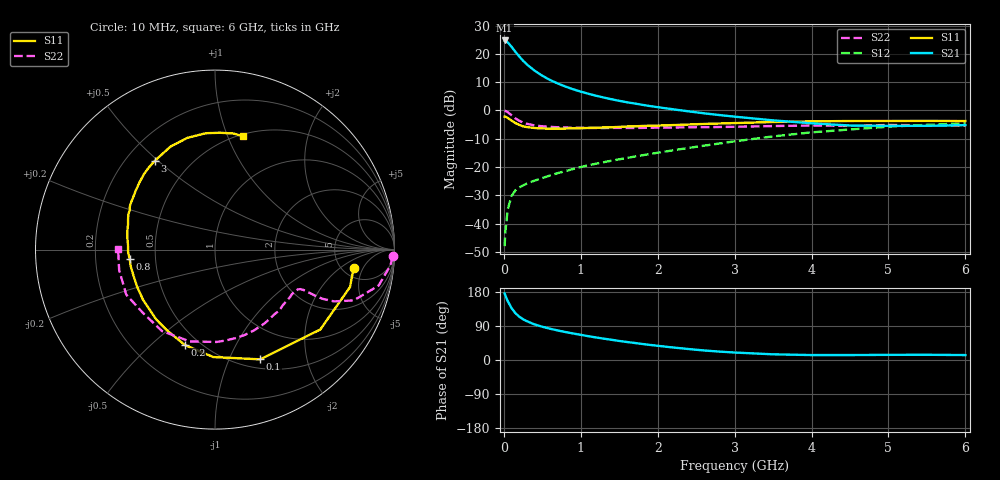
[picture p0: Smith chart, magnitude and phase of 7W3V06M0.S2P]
! Infineon Technologies  Discrete & RF Semiconductors
! BFS17W
! Si NPN RF Bipolar Junction Transistor in SOT323
! VCE = 3 V  IC = 6 mA
! Common Emitter S-Parameters:  August  1999
# GHz  S  MA  R  50
!  f  S11  S21  S12  S22
! GHz  MAG  ANG  MAG  ANG  MAG  ANG  MAG  ANG
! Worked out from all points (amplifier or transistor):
!   36 points, 10 MHz to 6 GHz, reference 50 ohm
!   highest |S21| = 24.7 dB at 10 MHz (marker M1)
!   |S21| within 3 dB of that: start of sweep to 121.7 MHz
!   unconditionally stable (mu >= 1): 499.1 MHz to 2.805 GHz; 4.255 GHz to end of sweep
!   at 250 MHz: K = 0.65, MSG = 22.0 dB, |S12| = -26.5 dB
!   at 1.4 GHz: K = 1.24, MAG = 7.9 dB, |S12| = -17.8 dB
!   at 6 GHz: K = 1.08, MAG = -2.1 dB, |S12| = -4.5 dB
!   S11 on the Smith chart (normalised r, x): 10 MHz: 6.29, -3.30; 100 MHz: 0.60, -1.31; 200 MHz: 0.42, -0.64; 800 MHz: 0.35, -0.05; 3 GHz: 0.32, +0.49; 6 GHz: 0.52, +1.14
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0.01  0.7791 -7.6  17.24 175.4  0.004 79.9  0.9921 -2.2
0.02  0.7807 -15.5  17.04 169.9  0.0072 85.0  0.9805 -5.3
0.05  0.7365 -37.2  16.02 155.6  0.0178 73.5  0.9333 -12.4
0.1  0.6613 -67.6  13.33 137.1  0.0307 60.7  0.8235 -20.1
0.15  0.5986 -91.0  10.88 123.6  0.0387 53.4  0.7237 -23.5
0.2  0.5571 -107.6  8.994 114.4  0.0435 51.5  0.6583 -24.6
0.25  0.5242 -120.3  7.559 107.6  0.0475 49.0  0.6105 -24.7
0.3  0.5082 -130.2  6.491 102.3  0.0511 49.3  0.5813 -24.6
0.4  0.4889 -145.1  5.043 93.9  0.0576 50.7  0.543 -24.5
0.5  0.4805 -154.8  4.104 87.8  0.0638 52.9  0.5248 -24.8
0.6  0.4767 -162.6  3.453 82.6  0.0709 54.7  0.513 -25.6
0.8  0.4783 -173.9  2.646 73.8  0.0847 57.7  0.4991 -28.6
0.9  0.4845 -178.4  2.368 70.0  0.0923 59.4  0.4949 -30.4
1.1  0.4905 173.6  1.969 62.7  0.1076 61.0  0.4919 -34.6
1.3  0.5009 166.7  1.69 56.3  0.1221 62.3  0.4888 -39.6
1.6  0.5212 158.0  1.395 47.5  0.1446 63.7  0.4895 -47.3
2.2  0.5512 143.1  1.047 33.0  0.1977 65.5  0.5001 -64.5
3  0.5981 124.0  0.777 19.7  0.2843 63.4  0.5146 -89.0
3.5  0.6254 113.3  0.668 15.0  0.3482 59.6  0.5304 -105.3
4.5  0.6505 94.6  0.542 13.0  0.4611 47.4  0.5345 -138.8
5.5  0.6549 81.0  0.535 13.8  0.5565 35.0  0.5461 -167.9
6  0.6499 76.0  0.55 13.0  0.5939 29.0  0.5401 179.5
